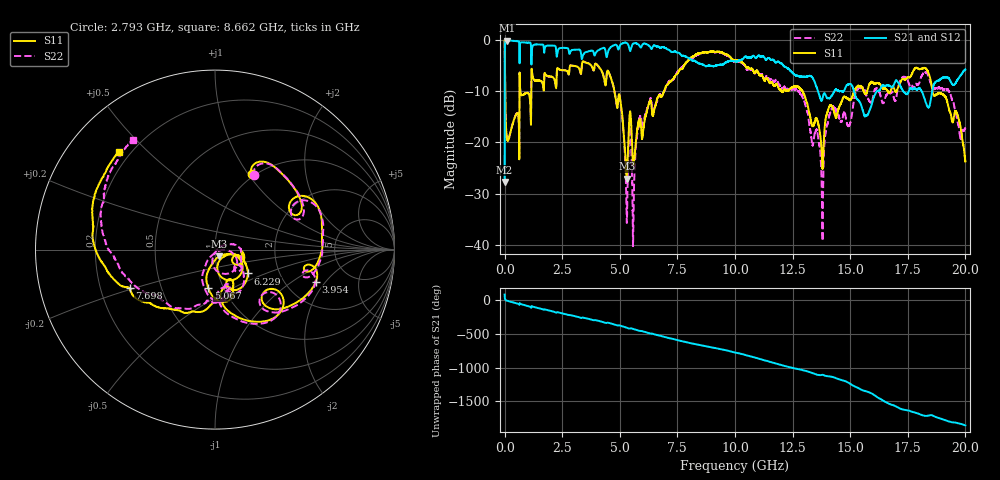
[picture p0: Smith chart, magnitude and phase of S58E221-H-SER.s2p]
!{S58E221}
!Johanson Technology Inc.
!www.johansontechnology.com
!Test Board Conditions:
!Substrate Type  RO4350B
!Substrate Thickness  60 mil
!Substrate Dk  3.66
!TL Type: GCPW
!TL Trace Width  115 mil
!TL Gap  52 mil
!Electrode orientation  Horizontal
!DUT TOPOLOGY	SERIES
!Mounting Pad LxW  55x428 mil
! Created Wed Apr 14 11:31:35 2021
# mhz S ma R 50
! 2 Port Network Data from SP1.SP block
! freq  magS11  angS11  magS21  angS21  magS12  angS12  magS22  angS22
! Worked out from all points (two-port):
!   20001 points, 300 kHz to 20 GHz, reference 50 ohm
!   highest |S21| = -0.06 dB at 100.3 MHz (marker M1); lowest = -27.7 dB at 300 kHz (marker M2)
!   |S21| within 3 dB of the highest: 1.175 GHz to 2.256 GHz (1.081 GHz wide, 63 % of centre); 4.448 GHz to 7.773 GHz (3.325 GHz wide, 54.4 % of centre)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
!   lowest |S11| = -27.1 dB at 5.301 GHz (marker M3), VSWR 1.09, Z = 52.4 - j3.87 ohm
!   |S11| at or under -10 dB: 4.771 GHz to 6.924 GHz (2.152 GHz wide, 36.8 % of centre); 12.93 GHz to 15.17 GHz (2.242 GHz wide, 16 % of centre); 18.57 GHz to end of sweep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
!   |S22| runs from -40.3 to -0.1 dB; largest |S21 - S12| = 0.012
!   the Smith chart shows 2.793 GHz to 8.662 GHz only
!   S11 on the Smith chart (normalised r, x): 2.793 GHz: 0.96, +1.04; 3.954 GHz: 2.92, -1.60; 5.067 GHz: 0.85, -0.38; 6.229 GHz: 1.39, -0.39; 7.698 GHz: 0.33, -0.19; 8.662 GHz: 0.16, +0.41
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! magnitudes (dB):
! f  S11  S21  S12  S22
! 300 kHz  0.0  -27.7  -27.6  -0.1
! 100.3 MHz  -19.2  -0.1  -0.1  -19.1
! 2.793 GHz  -6.6  -2.3  -2.3  -6.6
! 3.334 GHz  -6.0  -3.3  -3.3  -6.0
! 3.954 GHz  -4.6  -2.5  -2.5  -4.6
! 5.067 GHz  -13.2  -0.7  -0.7  -13.5
! 5.301 GHz  -27.1  -0.5  -0.5  -35.3
! 5.441 GHz  -14.0  -2.1  -2.1  -16.1
! 5.615 GHz  -23.8  -0.6  -0.6  -29.2
! 5.819 GHz  -15.7  -0.9  -0.9  -16.6
! 6.229 GHz  -12.9  -1.0  -1.0  -12.9
! 6.667 GHz  -11.1  -1.2  -1.2  -11.4
! 7.698 GHz  -5.6  -3.0  -3.0  -5.3
! 8.662 GHz  -2.4  -4.9  -4.9  -2.3
! 10 GHz  -4.0  -4.2  -4.2  -4.3
! 12.73 GHz  -9.1  -7.0  -6.8  -10.0
! 13.33 GHz  -16.5  -7.2  -7.2  -19.8
! 13.78 GHz  -23.4  -11.7  -11.6  -31.8
! 14.22 GHz  -12.9  -10.7  -10.8  -13.0
! 16.67 GHz  -10.2  -8.8  -8.9  -10.2
! 18.28 GHz  -5.5  -12.2  -12.1  -6.3
! 20 GHz  -23.7  -5.8  -5.7  -17.4
